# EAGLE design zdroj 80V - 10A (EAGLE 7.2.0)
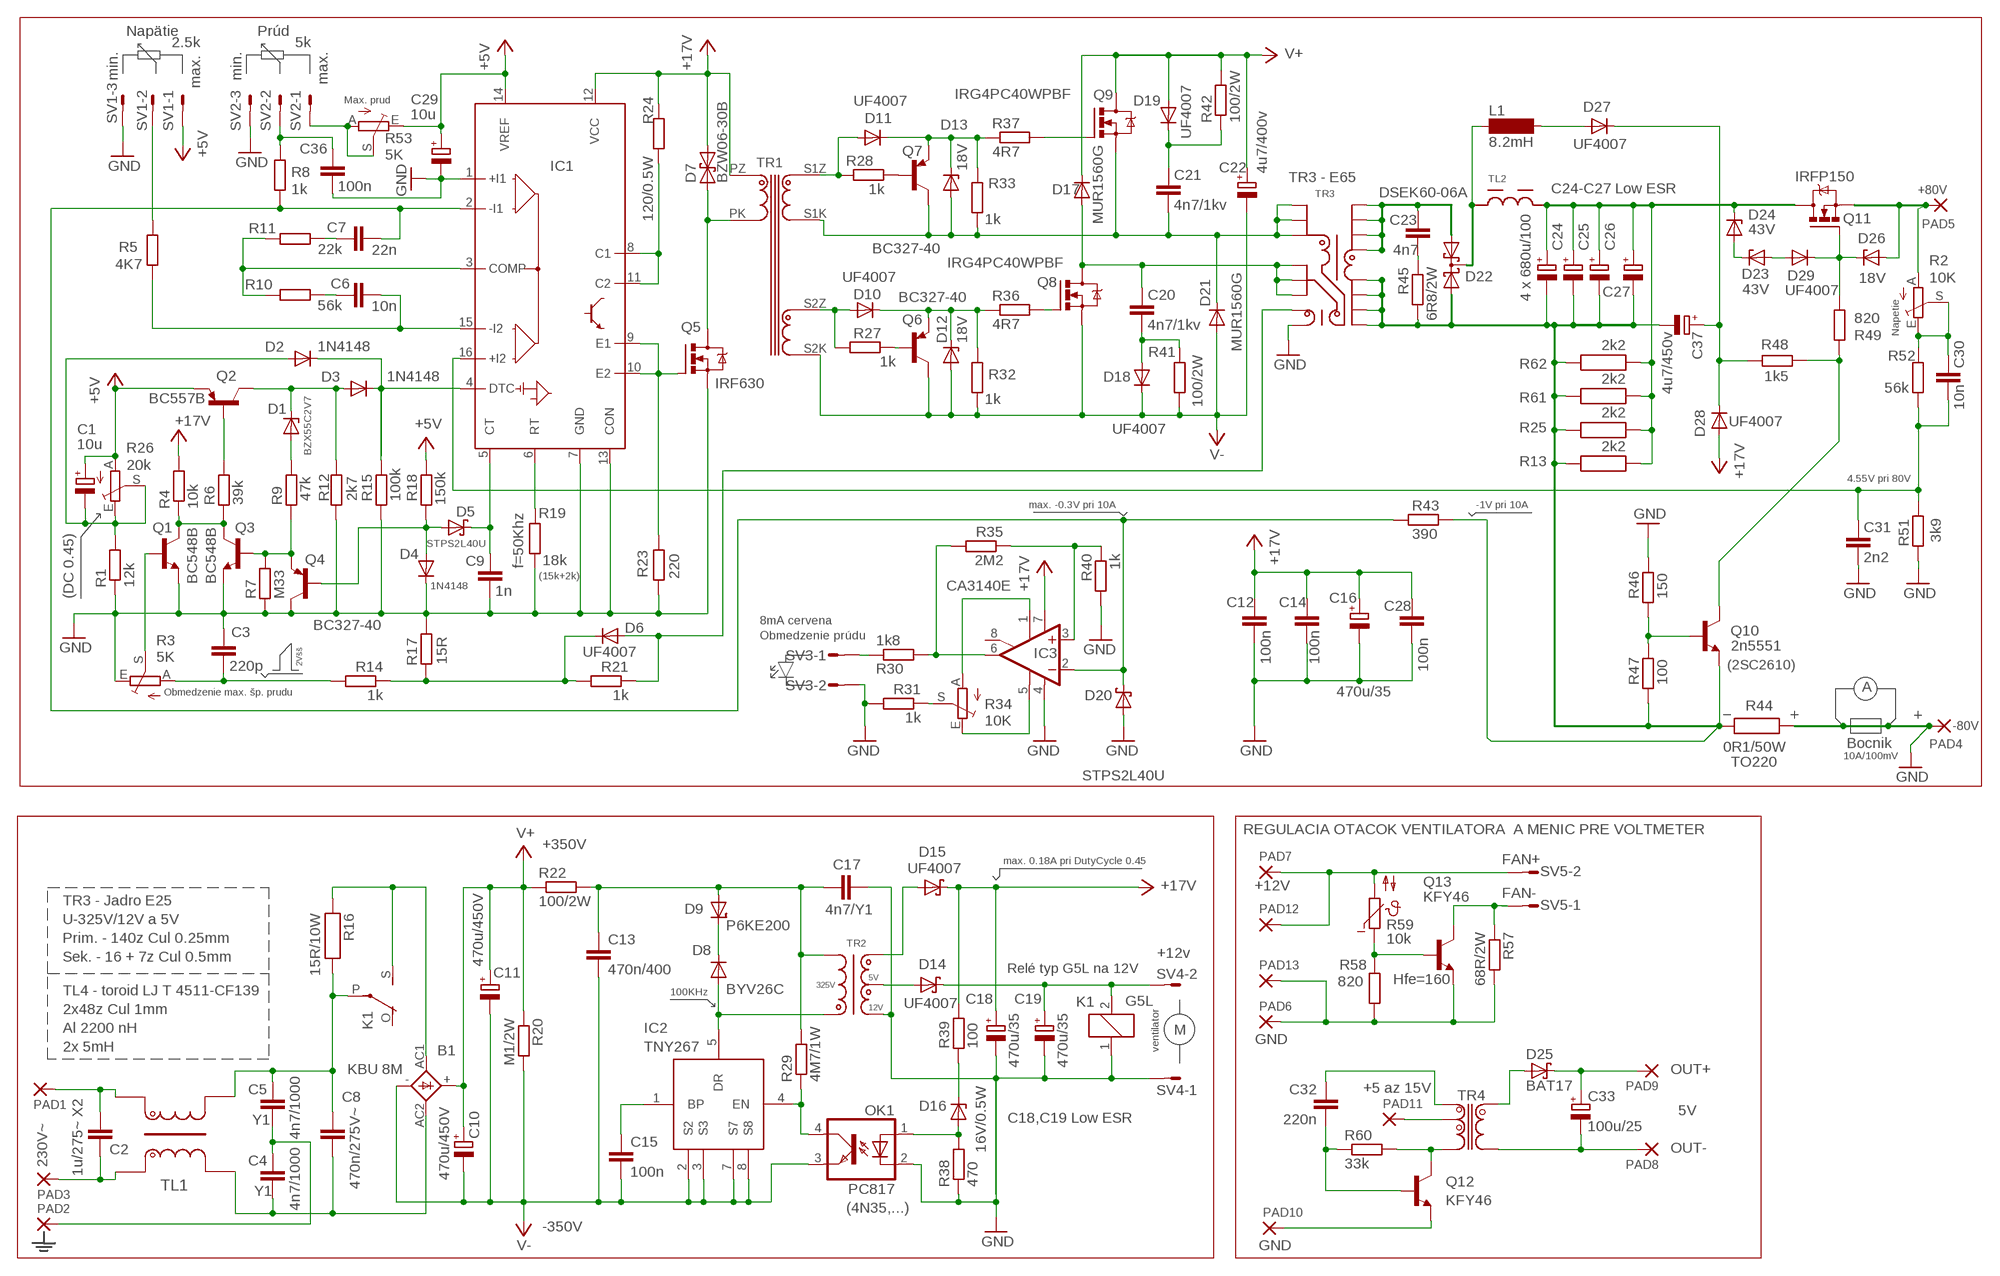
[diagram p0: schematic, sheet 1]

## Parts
B1  KBU 8M  KBU  [KBU]
C1  10u  CPOL-EUE5-4  [E5-4]
C2  1u/275~ X2  C-EU275-134X316  [C275-134X316]
C3  220p  C-EU050-024X044  [C050-024X044]
C4  4n7/1000  C-EU075-032X103  [C075-032X103]
C5  4n7/1000  C-EU075-032X103  [C075-032X103]
C6  10n  C-EU075-032X103  [C075-032X103]
C7  22n  C-EU050-024X044  [C050-024X044]
C8  470n/275V~  FOLIOVYRM22,5/10-26,5  [FOLIOVY_RM22,5/10-26,5]
C9  1n  C-EU050-024X044  [C050-024X044]
C10  470u/450V  CPOL-EUE10-30  [EB30D]
C11  470u/450V  CPOL-EUE10-30  [EB30D]
C12  100n  C-EU050-024X044  [C050-024X044]
C13  470n/400  C-EU225-087X268  [C225-087X268]
C14  100n  C-EU050-024X044  [C050-024X044]
C15  100n  C-EU050-024X044  [C050-024X044]
C16  470u/35  CPOL-EUE5-10.5  [E5-10,5]
C17  4n7/Y1  C-EU075-032X103  [C075-032X103]
C18  470u/35  CPOL-EUE5-10.5  [E5-10,5]
C19  470u/35  CPOL-EUE5-10.5  [E5-10,5]
C20  4n7/1kv  C-EU050-024X044  [C050-024X044]
C21  4n7/1kv  C-EU050-024X044  [C050-024X044]
C22  4u7/400v  CPOL-EUE5-10.5  [E5-10,5]
C23  4n7  C-EU050-024X044  [C050-024X044]
C24  CPOL-EUE7.5-18  [E7,5-18]
C25  CPOL-EUE7.5-18  [E7,5-18]
C26  CPOL-EUE7.5-18  [E7,5-18]
C27  4 x 680u/100  CPOL-EUE7.5-18  [E7,5-18]
C28  100n  C-EU050-024X044  [C050-024X044]
C29  10u  CPOL-EUE2.5-5  [E2,5-5]
C30  10n  C-EU075-032X103  [C075-032X103]
C31  2n2  C-EU050-024X044  [C050-024X044]
C32  220n  C-EU050-024X044  [C050-024X044]
C33  100u/25  CPOL-EUE2.5-6  [E2,5-6]
C36  100n  C-EU050-024X044  [C050-024X044]
C37  4u7/450v  CPOL-EUE5-10.5  [E5-10,5]
D1  BZX55C2V7  ZENER-DIODEDO34-7  [DO34Z7]
D2  1N4148  1N4148DO35-7  [DO35-7]
D3  1N4148  1N4148DO35-7  [DO35-7]
D4  1N4148  1N4148DO35-10  [DO35-10]
D5  STPS2L40U  BAT19  [DO35-10]
D6  UF4007  1N4004  [DO41-10]
D7  BZW06-30B  ZZ22  [P2-15]
D8  BYV26C  DIODE-D-7.5  [D-7.5]
D9  P6KE200  DIODE-DO204-10  [DO204-10]
D10  UF4007  1N4148DO35-7  [DO35-7]
D11  UF4007  1N4148-12  [DO35-12]
D12  18V  BZX90  [DO34Z7]
D13  18V  BZX90  [DO34Z7]
D14  UF4007  BAT49  [DO41-10]
D15  UF4007  BAT49  [DO41-10]
D16  16V/0.5W  BZX90  [DO34Z7]
D17  MUR1560G  BYW29  [DO220S]
D18  UF4007  1N4004  [DO41-10]
D19  UF4007  1N4007-12  [DO41-12]
D20  STPS2L40U  BAT19  [DO35-10]
D21  MUR1560G  BYW29  [DO220S]
D22  DSEK60-06A  DIODE_2SCHOTTKY-SOT93V  [SOT93S]
D23  43V  BZX90  [DO34Z7]
D24  43V  BZX90  [DO34Z7]
D25  BAT17  BAT19  [DO35-10]
D26  18V  BZX85  [DO41Z10]
D27  UF4007  DIODE-DO34-7  [DO34-7]
D28  UF4007  DIODE-DO34-7  [DO34-7]
D29  UF4007  DIODE-DO34-7  [DO34-7]
IC1  TL494  [DIL16]
IC2  TNY267  [DIL7]
IC3  CA3140E  OP07N  [DIL08]
K1  G5L  [G5LE]
L1  8.2mH  SD12K100  [SD12K100]
OK1  PC817  [DIL04]
PAD1  2,54/1,0  [2,54/1,0]
PAD2  2,54/1,0  [2,54/1,0]
PAD3  2,54/1,0  [2,54/1,0]
PAD4  -80V  3,81/1,4  [3,81/1,4]
PAD5  +80V  3,81/1,4  [3,81/1,4]
PAD6  2,54/0,8  [2,54/0,8]
PAD7  2,54/0,8  [2,54/0,8]
PAD8  2,54/0,8  [2,54/0,8]
PAD9  2,54/0,8  [2,54/0,8]
PAD10  2,54/0,8  [2,54/0,8]
PAD11  2,54/0,8  [2,54/0,8]
PAD12  2,54/0,8  [2,54/0,8]
PAD13  2,54/0,8  [2,54/0,8]
Q1  BC548B  BC338  [TO92-EBC]
Q2  BC557B  [TO92-EBC]
Q3  BC548B  BC338  [TO92-EBC]
Q4  BC327-40  [TO92-EBC]
Q5  IRF630  IRF540  [TO220BV]
Q6  BC327-40  BC327  [TO92-EBC]
Q7  BC327-40  BC327  [TO92-EBC]
Q8  IRG4PC40WPBF  IRFPC40  [TO247BV]
Q9  IRG4PC40WPBF  IRFPC40  [TO247BV]
Q10  2n5551  29-NPN-TO92-EBC  [TO92-EBC]
Q11  IRFP150  IRFPC40  [TO247BV]
Q12  KFY46  2N1711  [TO39]
Q13  KFY46  2N1711  [TO39]
R1  12k  R-EU_0207/7  [0207/7]
R2  10K  B64YW  [B64YW]
R3  5K  B64YW  [B64YW]
R4  10k  R-EU_0207/10  [0207/10]
R5  4K7  R-EU_0207/7  [0207/7]
R6  39k  R-EU_0207/7  [0207/7]
R7  M33  R-EU_0207/7  [0207/7]
R8  1k  R-EU_0207/7  [0207/7]
R9  47k  R-EU_0207/7  [0207/7]
R10  56k  R-EU_0207/10  [0207/10]
R11  22k  R-EU_0207/7  [0207/7]
R12  2k7  R-EU_0207/10  [0207/10]
R13  2k2  R5W  [R5W]
R14  1k  R-EU_0207/10  [0207/10]
R15  100k  R-EU_0207/10  [0207/10]
R16  15R/10W  RMNS-10  [RMNS-10]
R17  15R  R-EU_0207/10  [0207/10]
R18  150k  R-EU_0207/7  [0207/7]
R19  18k  R-EU_0207/7  [0207/7]
R20  M1/2W  R-EU_0817/7V  [P0817V]
R21  1k  R-EU_0207/10  [0207/10]
R22  100/2W  R-EU_0411/15  [0411/15]
R23  220  R-EU_0207/10  [0207/10]
R24  120/0.5W  R-EU_0207/7  [0207/7]
R25  2k2  R5W  [R5W]
R26  20k  B64YW  [B64YW]
R27  1k  R-EU_0207/7  [0207/7]
R28  1k  R-EU_0207/12  [0207/12]
R29  4M7/1W  R-EU_0207/10  [0207/10]
R30  1k8  R-EU_0207/7  [0207/7]
R31  1k  R-EU_0207/7  [0207/7]
R32  1k  R-EU_0207/7  [0207/7]
R33  1k  R-EU_0207/7  [0207/7]
R34  10K  B64YW  [B64YW]
R35  2M2  R-EU_0207/7  [0207/7]
R36  4R7  R-EU_0207/7  [0207/7]
R37  4R7  R-EU_0207/7  [0207/7]
R38  470  R-EU_0207/10  [0207/10]
R39  100  R-EU_0207/7  [0207/7]
R40  1k  R-EU_0207/7  [0207/7]
R41  100/2W  R-EU_0411/12  [0411/12]
R42  100/2W  R-EU_0411/12  [0411/12]
R43  390  R-EU_0207/12  [0207/12]
R44  0R1/50W  RMNS-10  [RMNS-10]
R45  6R8/2W  R-EU_0309/12  [0309/12]
R46  150  R-EU_0207/10  [0207/10]
R47  100  R-EU_0207/10  [0207/10]
R48  1k5  R-EU_0207/10  [0207/10]
R49  820  R-EU_0207/10  [0207/10]
R51  3k9  R-EU_0207/7  [0207/7]
R52  56k  R-EU_0207/10  [0207/10]
R53  5K  B64YW  [B64YW]
R57  68R/2W  R-EU_0309/10  [0309/10]
R58  820  R-EU_0207/10  [0207/10]
R59  10k  NTC640  [P640]
R60  33k  R-EU_0207/7  [0207/7]
R61  2k2  R5W  [R5W]
R62  2k2  R5W  [R5W]
SV1  S03P  [S03P]
SV2  S03P  [S03P]
SV3  S02P  [S02P]
SV4  S02P  [S02P]
SV5  S02P  [S02P]
TL1  TR-F  [TR-F]
TL2  TL-TOR20/45  [TL-TOR-40/48]
TR1  TR2  [TR2]
TR2  TR4  [TR4]
TR3  TR1-E65-2  [TR1-E65-2]
TR4  TR-X1  [TR-X1]

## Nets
+5V: C1.+ C29.+ IC1.14(VREF) Q2.E R18.1 R26.A R53.E SV1.1
+17V: C12.1 C14.1 C16.+ C18.+ C28.1 D7.C D15.C D28.A IC1.12(VCC) IC3.7(V+) R4.2 R24.1 R39.2 TR1.PZ
GND: C3.2 C9.1 C12.2 C14.2 C16.- C17.2 C18.- C19.- C28.2 C29.- C31.2 C36.2 D4.C D20.A IC1.1(+I1) IC1.7(GND) IC1.13(CON) IC3.4(V-) K1.1 OK1.2(C) PAD4.1(P) Q1.E Q3.E Q4.C Q5.S R1.1 R3.E R7.2 R12.1 R15.1 R17.1 R19.1 R23.2 R31.2 R38.1 R40.2 R44.2 R46.2 R51.1 SV1.3 SV2.3 SV3.2 SV4.1 TR2.P3 TR3.1
N$1: C2.1 PAD3.1(P) TL1.A1
N$2: C2.2 PAD1.1(P) TL1.B1
N$3: C5.1 C8.P$1 K1.P(2:P) R16.2 TL1.B2
N$4: C13.1 C17.1 D9.A R22.2 R29.2 TR2.P1
N$5: C19.+ D14.C K1.2 SV4.2
N$6: B1.AC1 K1.S(2:S) R16.1
N$7: D2.C D3.C IC1.4(DTC) R15.2
N$8: D14.A TR2.P4
N$9: D27.A L1.2
N$10: IC1.9(E1) IC1.10(E2) Q5.G R23.1
N$11: D26.C D29.C Q11.G R49.2
N$13: IC3.3(+IN) R35.1 R40.1
N$14: D26.A PAD5.1(P) Q11.S R2.A
N$15: D8.C D9.C
N$16: C30.1 R2.E R2.S R52.1
N$17: C30.2 C31.1 IC1.16(+I2) R51.2 R52.2
N$18: C9.2 D5.C IC1.5(CT)
N$19: IC1.6(RT) R19.2
N$20: D6.C R14.1 R17.2 R21.2
N$21: D6.A R21.1 TR3.2
N$22: IC1.8(C1) IC1.11(C2) R24.2
N$23: D7.A Q5.D TR1.PK
N$24: Q7.B R28.2
N$25: D23.C D24.A
N$26: D11.A R28.1 TR1.S1Z
N$27: D11.C D13.C Q7.E R33.1 R37.1
N$28: Q6.B R27.2
N$29: D10.A R27.1 TR1.S2Z
N$30: C21.2 D13.A D21.C Q7.C Q9.S R33.2 TR1.S1K TR3.6 TR3.7 TR3.8
N$31: D10.C D12.C Q6.E R32.1 R36.1
N$32: B1.AC2 C4.2 C8.P$2 TL1.A2
N$33: D8.A IC2.5(DR) TR2.P2
N$34: C15.1 IC2.1(BP)
N$35: IC2.4(EN) OK1.4(COL) R29.1
N$36: D22.C L1.1 TL2.2
N$37: D15.A TR2.P5
N$38: Q8.G R36.2
N$39: C20.2 D17.A Q8.D TR3.3 TR3.4 TR3.5
N$40: D16.A OK1.1(A) R38.2
N$41: D16.C R39.1
N$42: Q9.G R37.2
N$43: C1.- D2.A R1.2 R26.E R26.S
N$44: C20.1 D18.A R41.1
N$45: C21.1 D19.C R42.1
N$46: IC3.6(OUT) R30.2 R35.2
N$47: C23.2 D22.A2 TR3.9 TR3.10 TR3.11 TR3.12
N$48: C24.+ C25.+ C26.+ C27.+ D24.C Q11.D R13.1 R25.1 R61.1 R62.1 TL2.1
N$49: C7.2 D20.C IC1.2(-I1) IC3.2(-IN) R8.2 R43.1
N$50: D1.C D3.A Q2.C R12.2
N$51: C24.- C25.- C26.- C27.- C37.- D22.A1 Q10.E R13.2 R25.2 R43.2 R44.1 R45.2 R47.1 R61.2 R62.2 TR3.13 TR3.14 TR3.15 TR3.16
N$52: R53.A R53.S SV2.1
N$53: C36.1 R8.1 SV2.2
N$54: C6.2 IC1.15(-I2) R5.1
N$55: R5.2 SV1.2
N$56: Q10.B R46.1 R47.2
N$57: PAD7.1(P) PAD12.1(P) R59.2 SV5.2
N$58: C6.1 R10.2
N$59: Q2.B R6.1
N$60: PAD6.1(P) PAD13.1(P) Q13.1(E) R57.2 R58.1
N$61: Q1.C Q3.C R4.1 R6.2
N$62: Q13.3(C) R57.1 SV5.1
N$63: Q3.B Q4.E R7.1 R9.2
N$64: IC3.5(OPT) R34.E
N$65: IC3.1(ON1) R34.A
N$66: IC1.3(COMP) R10.1 R11.1
N$67: Q10.C R48.2 R49.1
N$68: R31.1 R34.S
N$69: C7.1 R11.2
N$70: C37.+ D27.C D28.C R48.1
N$71: C3.1 R3.A R14.2
N$72: C4.1 C5.2 PAD2.1(P)
N$73: Q1.B R3.S
N$74: R30.1 SV3.1
N$75: Q13.2(B) R58.2 R59.1
N$76: C32.2 Q12.2(B) R60.1
N$77: Q12.3(C) R60.2 TR4.P
N$78: C33.+ D25.C PAD9.1(P)
N$79: D1.A R9.1
N$80: D4.A D5.A Q4.B R18.2
N$81: C23.1 R45.1
N$82: C33.- PAD8.1(P) TR4.S2
N$83: C32.1 TR4.I(B)
N$84: PAD11.1(P) TR4.SP
N$85: PAD10.1(P) Q12.1(E)
N$86: D25.A TR4.S1
N$93: D23.A D29.A
V+: B1.+ C10.+ C11.+ C22.+ D17.C D19.A Q9.D R20.1 R22.1 R42.2
V-: B1.- C10.- C11.- C13.2 C15.2 C22.- D12.A D18.C D21.A IC2.2(S2) IC2.3(S3) IC2.7(S7) IC2.8(S8) OK1.3(EMIT) Q6.C Q8.S R20.2 R32.2 R41.2 TR1.S2K
Unconnected: IC3.8(ON2) K1.O(2:O)

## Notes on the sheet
- Napätie | Prúd
- min. | 2.5k | min. | 5k | max.
- max.
- Max. prud
- TR3 - E65
- C24-C27 Low ESR
- Napetie
- 4.55V pri 80V
- max. -0.3V pri 10A | -1V pri 10A
- f=50Khz
- (15k+2k)
- (DC 0.45)
- 8mA cervena
- Obmedzenie prúdu
- 2Všš
- (2SC2610)
- A
- Obmedzenie max. šp. prudu
- Bocnik
- 10A/100mV
- TO220
- REGULACIA OTACOK VENTILATORA  A MENIC PRE VOLTMETER
- +350V
- max. 0.18A pri DutyCycle 0.45 | FAN+
- +12V
- FAN-
- TR3 - Jadro E25
- U-325V/12V a 5V
- Prim. - 140z Cul 0.25mm
- Sek. - 16 + 7z Cul 0.5mm | +12v
- Relé typ G5L na 12V
- 5V
- Hfe=160
- 325V
- TL4 - toroid LJ T 4511-CF139 | 100KHz
- 12V
- 2x48z Cul 1mm
- Al 2200 nH | M
- GND
- 2x 5mH | ventilator
- OUT+
- +5 az 15V
- 5V
- 230V~ | Y1 | C18,C19 Low ESR
- OUT-
- Y1
- (4N35,...)
- -350V
- GND

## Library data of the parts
B1 = rectifier:KBU: DIOTEC RECTIFIER
C1 C10 C11 C16 C18 C19 C22 C24-C27 C29 C33 C37 = rcl:CPOL-EU: POLARIZED CAPACITOR, European symbol
C2-C7 C9 C12-C15 C17 C20 C21 C23 C28 C30-C32 C36 = rcl:C-EU: CAPACITOR, European symbol
C8 = #Kondenzatory:FOLIOVY
D1 = diode:ZENER-DIODE: Z-Diode
D2-D4 D10 = diode:1N4148: DIODE
D5 D20 D25 = diode:BAT19: DIODE
D6 D18 = diode:1N4004: DIODE
D7 = diode:ZZ22: DIODE
D8 D9 D27-D29 = diode:DIODE-: DIODE
D11 = diode-1:1N4148-12
D12 D13 D16 D23 D24 = diode:BZX90: Z DIODE
D14 D15 = diode:BAT49: DIODE
D17 D21 = diode:BYW29: DIODE
D19 = UNIVERSAL:1N4007-12
D22 = diode-1:DIODE_2SCHOTTKY-: Dual SCHOTTKY DIODE common cathode
D26 = diode:BZX85: Z DIODE
IC1 = UNIVERSAL:TL494: TL494N upraveny pre priepustny menic. DIL16
IC2 = UNIVERSAL:TNY267; IC: TNY267
IC3 = linear:OP07*: OP AMP
K1 = relay:G5L: RELAY 1 x switch, 10 A/120 V AC, 8 A/30 V ADC, Omron
L1 = inductor-neosid:SD12: INDUCTOR; OC_FARNELL: unknown; OC_NEWARK: unknown
OK1 = optocoupler:PC817: SHARP OPTO COUPLER; MPN: PC817X4J000F; OC_FARNELL: 9707727; OC_NEWARK: 97K7059
PAD1-PAD3 = PLOSNE BODY:2,54/1,0
PAD4 PAD5 = PLOSNE BODY:3,81/1,4
PAD6-PAD13 = PLOSNE BODY:2,54/0,8
Q1 Q3 = transistor-npn:BC338*: NPN Transistor
Q2 = transistor-pnp:BC557*: PNP Transistror
Q4 Q6 Q7 = transistor-pnp:BC327*: PNP Transistror
Q5 = transistor-power:IRF540: HEXFET Power MOSFET
Q8 Q9 Q11 = transistor-power:IRFPC40: N-CHANNEL MOS FET
Q10 = transistor:*-NPN-: NPN Transistror BF959 corrected 2008.03.06
Q12 Q13 = transistor-npn:2N1711: NPN Transistor
R1 R4-R12 R14 R15 R17-R24 R27-R33 R35-R43 R45-R49 R51 R52 R57 R58 R60 = rcl:R-EU_: RESISTOR, European symbol
R2 R3 R26 R34 R53 = pot:B64YW
R13 R25 R61 R62 = UNIVERSAL:R5W
R16 R44 = UNIVERSAL:RMNS-10
R59 = ptc-ntc:NTC640: PHILIPS NTC; OC_FARNELL: unknown; OC_NEWARK: unknown
SV1 SV2 = con-amp-mt:S03P: AMP MT CONNECTOR; OC_FARNELL: unknown; OC_NEWARK: unknown
SV3-SV5 = con-amp-mt:S02P: AMP MT CONNECTOR; OC_FARNELL: unknown; OC_NEWARK: unknown
TL1 = UNIVERSAL:TR-F
TL2 = UNIVERSAL:TL-TOR20/45
TR1 = UNIVERSAL:TR2
TR2 = UNIVERSAL:TR4
TR3 = UNIVERSAL:TR1-E65-2: Trafo E65 s prehodenymi vyvodami.
TR4 = UNIVERSAL:TR-X1

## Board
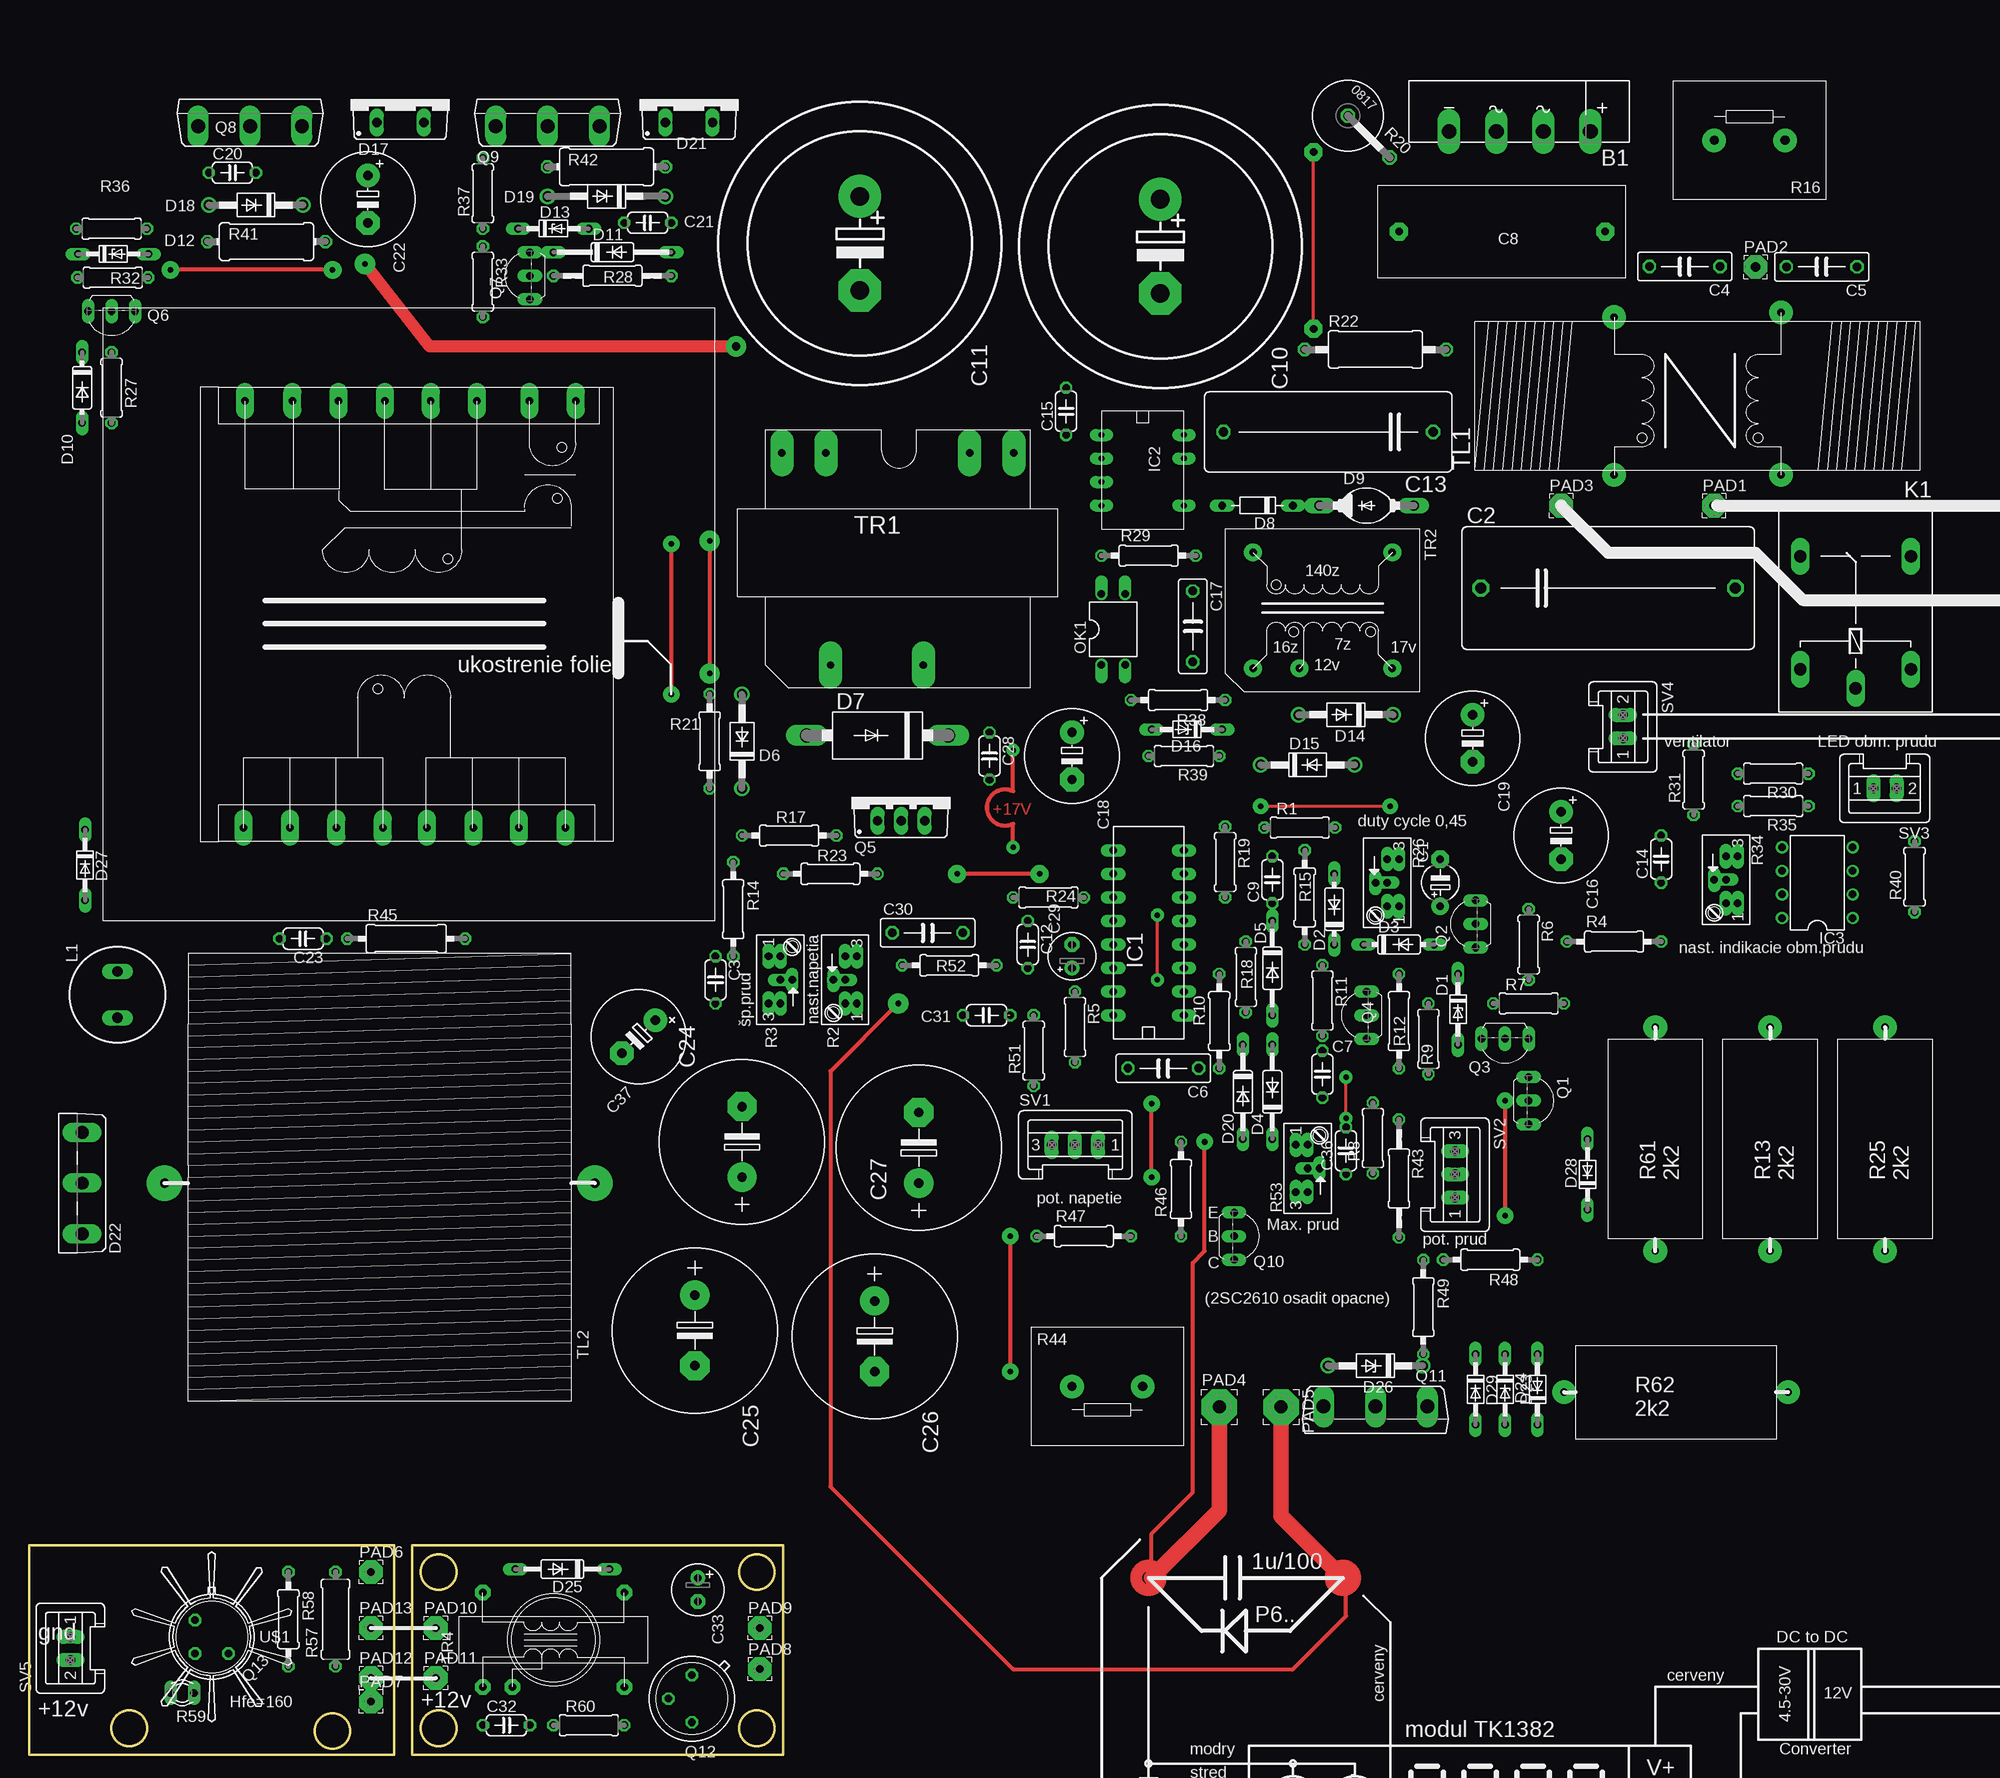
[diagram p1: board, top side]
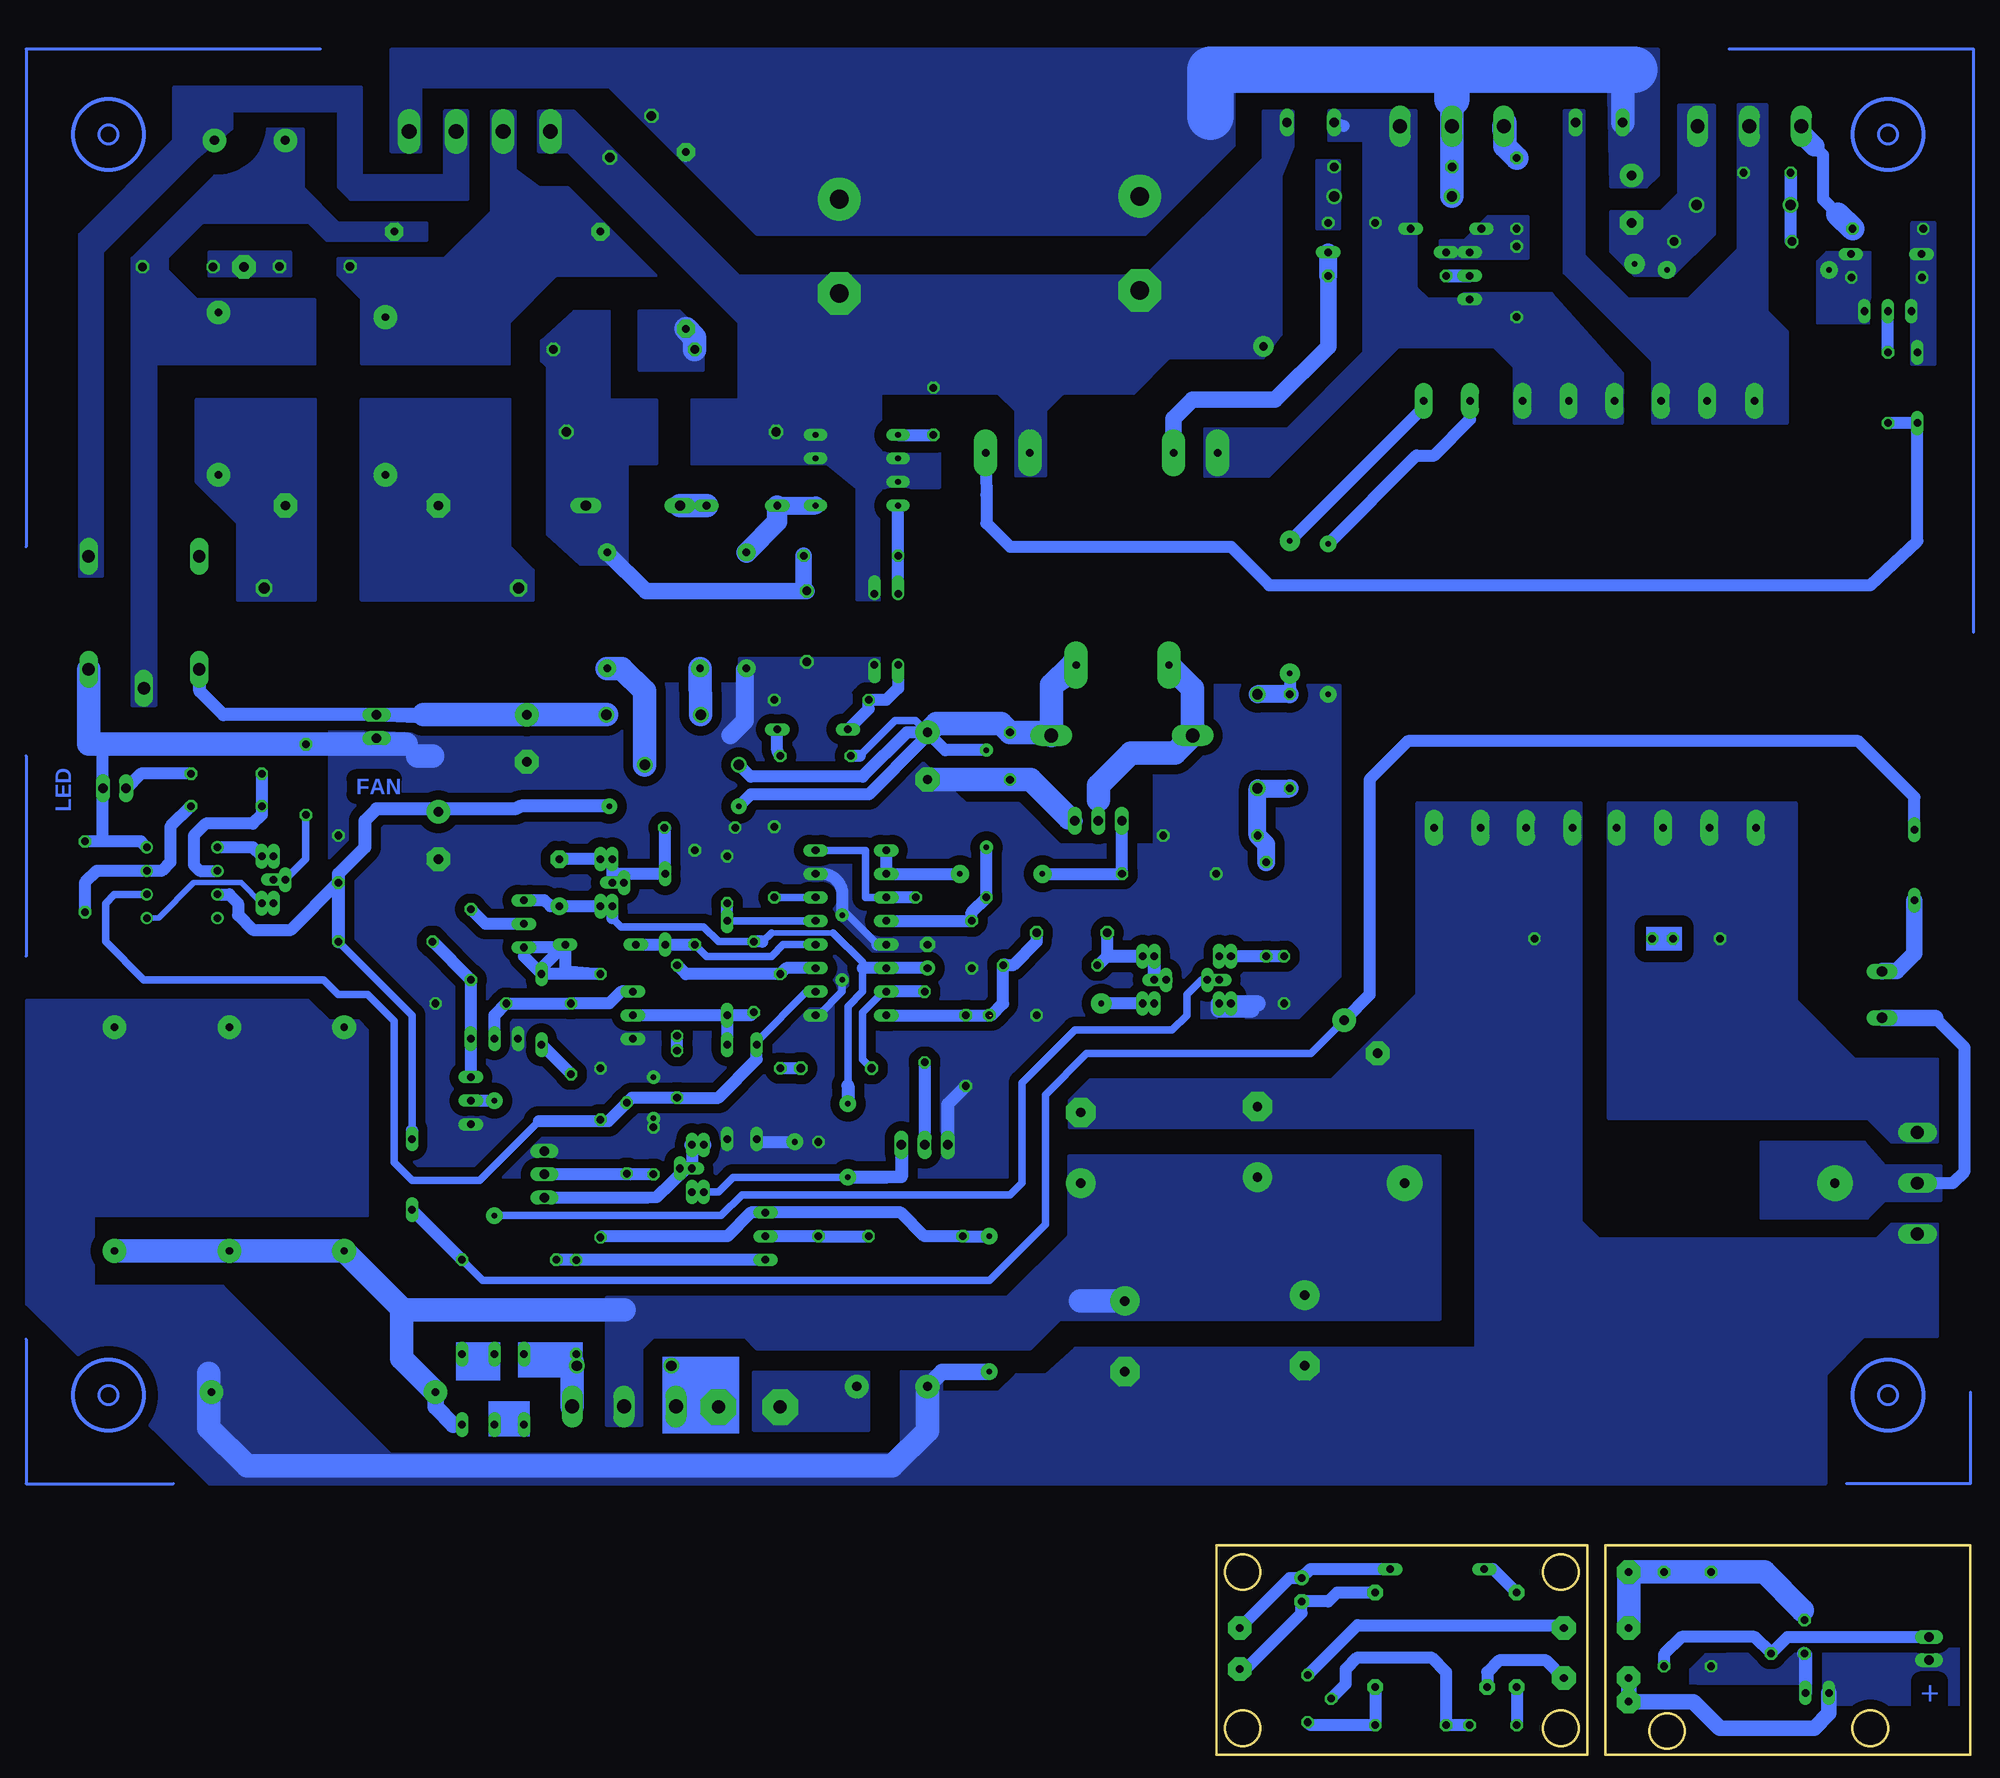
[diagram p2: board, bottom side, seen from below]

Size 81.28 x 22.54 mm. Coordinates in mm from the lower left corner, seen from the top.
Outline: 0,0 39.37,0 39.37,22.54 0,22.54 0,0
Outline: 41.27,0 41.27,22.54 81.28,22.54 81.28,0 41.27,0
Outline: circle at 10.79,2.86 radius 1.91
Outline: circle at 32.7,2.54 radius 1.91
Outline: circle at 44.13,2.86 radius 1.91
Outline: circle at 44.13,19.69 radius 1.91
Outline: circle at 78.42,19.69 radius 1.91
Outline: circle at 78.42,2.86 radius 1.91
Copper layers (1*16): Top 0.035mm / dielectric 1.5mm / Bottom 0.035mm
Design rules "default": minimum track width 10mil, minimum drill 24mil, track to track 8mil, track to pad 8mil, pad to pad 8mil, via to via 8mil, smd to smd 8mil, copper to edge 40mil, drill to drill 8mil, minimum pad ring 10mil, minimum via ring 8mil, stop-mask expansion 4mil, vias tented up to drill 0mil, thermal gap 10mil

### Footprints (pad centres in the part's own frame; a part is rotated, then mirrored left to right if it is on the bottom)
KBU = drill 1.6 long: + -7.62,2.54; - 7.62,2.54; AC1 -2.54,2.54; AC2 2.54,2.54
E5-4 = drill 0.813 pad 1.905: + -2.54,0 | drill 0.813 pad 1.905 octagon: - 2.54,0
C275-134X316 = drill 1.194 octagon: 1 -13.716,0; 2 13.716,0
C050-024X044 = drill 0.813 octagon: 1 -2.54,0; 2 2.54,0
C075-032X103 = drill 0.914 octagon: 1 -3.81,0; 2 3.81,0
FOLIOVY_RM22,5/10-26,5 = drill 0.8 pad 1.93 octagon: P$1 -11.113,0; P$2 11.113,0
EB30D = drill 2.007 pad 4.597: + -5.08,0 | drill 2.007 pad 4.597 octagon: - 5.08,0
C225-087X268 = drill 1.016 octagon: 1 -11.303,0; 2 11.303,0
E5-10,5 = drill 1.016 pad 2.54: + -2.54,0 | drill 1.016 pad 2.54 octagon: - 2.54,0
E7,5-18 = drill 1.016 pad 3.15: + -3.81,0 | drill 1.016 pad 3.15 octagon: - 3.81,0
E2,5-5 = drill 0.813 pad 1.6: + -1.27,0 | drill 0.813 pad 1.6 octagon: - 1.27,0
E2,5-6 = drill 0.813 pad 1.6: + -1.27,0 | drill 0.813 pad 1.6 octagon: - 1.27,0
DO34Z7 = drill 0.813 long: A 3.81,0; C -3.81,0
DO35-7 = drill 0.813 long: A 3.81,0; C -3.81,0
DO35-10 = drill 0.813 long: A 5.08,0; C -5.08,0
DO41-10 = drill 1.118: A 5.08,0; C -5.08,0
P2-15 = drill 1.499 long: A 7.62,0; C -7.62,0
D-7.5 = drill 0.813 long: A 3.81,0; C -3.81,0
DO204-10 = drill 1.118 long: A 5.08,0; C -5.08,0
DO35-12 = drill 0.813 long: A 6.35,0; C -6.35,0
DO220S = drill 1.016 long: A 2.54,-2.54; C -2.54,-2.54
DO41-12 = drill 1.118: A 6.35,0; C -6.35,0
SOT93S = drill 1.397 long: A1 -5.461,-2.54; A2 5.461,-2.54; C 0,-2.54
DO41Z10 = drill 1.118: A 5.08,0; C -5.08,0
DO34-7 = drill 0.813 long: A 3.81,0; C -3.81,0
DIL16 = drill 0.813 pad 1.27 long: 1 0,1.27; 2 2.54,1.27; 3 5.08,1.27; 4 7.62,1.27; 5 10.16,1.27; 6 12.7,1.27; 7 15.24,1.27; 8 17.78,1.27; 9 17.78,8.89; 10 15.24,8.89; 11 12.7,8.89; 12 10.16,8.89; 13 7.62,8.89; 14 5.08,8.89; 15 2.54,8.89; 16 0,8.89
DIL7 = drill 0.61 pad 1.27 long: 1 2.54,0; 2 5.08,0; 3 7.62,0; 4 10.16,0; 5 10.16,8.89; 7 5.08,8.89; 8 2.54,8.89
DIL08 = drill 0.813 pad 1.27: 1 -3.81,-3.81; 2 -1.27,-3.81; 3 1.27,-3.81; 4 3.81,-3.81; 5 3.81,3.81; 6 1.27,3.81; 7 -1.27,3.81; 8 -3.81,3.81
G5LE = drill 1.321 long: 1 -7.493,-5.969; 2 -7.493,5.969; O 4.699,5.969; P -9.525,0; S 4.699,-5.969
SD12K100 = drill 1.1 long: 1 -2.5,0; 2 2.5,0
DIL04 = drill 0.813 offset: 1 -1.27,-3.81; 2 1.27,-3.81; 3 1.27,3.81; 4 -1.27,3.81
2,54/1,0 = drill 1.016 pad 2.54 octagon: 1 0,0
3,81/1,4 = drill 1.397 pad 3.81 octagon: 1 0,0
2,54/0,8 = drill 0.813 pad 2.54 octagon: 1 0,0
TO92-EBC = drill 0.813 long: B 0,-1.27; C -2.54,-1.27; E 2.54,-1.27
TO220BV = drill 1.016 long: D 0,-2.54; G -2.54,-2.54; S 2.54,-2.54
TO247BV = drill 1.499 long: D 0,-2.921; G -5.588,-2.921; S 5.588,-2.921
TO92-EBC' = drill 0.813 long: B 0,-1.27; C 2.54,-1.27; E -2.54,-1.27
TO39 = drill 0.813 octagon: 1 0,-2.54; 2 2.54,0; 3 0,2.54
0207/7 = drill 0.813 octagon: 1 -3.81,0; 2 3.81,0
B64YW = drill 0.813 long: A 2.54,0; A1 2.54,1.27; E -2.54,0; E1 -2.54,1.27; S 0,0; S1 0,-1.27 | drill 0.813 octagon: S2 0,-1.27
0207/10 = drill 0.813 octagon: 1 -5.08,0; 2 5.08,0
R5W = drill 0.8 pad 2.54: 1 1.27,0; 2 25.4,0
RMNS-10 = drill 1 pad 2.54: 1 4.445,6.35; 2 12.065,6.35
P0817V = drill 1.016 octagon: 1 -5.08,0; 2 1.27,0
0411/15 = drill 0.914 octagon: 1 -7.62,0; 2 7.62,0
0207/12 = drill 0.813 octagon: 1 -6.35,0; 2 6.35,0
0411/12 = drill 0.914 octagon: 1 -6.35,0; 2 6.35,0
0309/12 = drill 0.813 octagon: 1 -6.35,0; 2 6.35,0
0309/10 = drill 0.813 octagon: 1 -5.08,0; 2 5.08,0
P640 = drill 0.813 long: 1 -1.27,0; 2 1.27,0
S03P = drill 1.016 long: 1 2.5,0; 2 0,0; 3 -2.5,0
S02P = drill 1.016 long: 1 1.25,0; 2 -1.25,0
TR-F = drill 0.8 pad 2.54: A1 -0.5,33; A2 16.5,33; B1 -0.5,15; B2 17,15
TL-TOR-40/48 = drill 1 pad 3.81: 1 -2.54,24.765; 2 43.815,24.765
TR2 = drill 0.8 pad 2.54 long: PK 7,3.135; PZ 17,3.135; S1K 1.75,26; S1Z 6.5,26; S2K 22,26; S2Z 26.75,26
TR4 = drill 0.8 pad 1.93: P1 2.5,18; P2 2.5,3; P3 15,3; P4 15,8; P5 15,18
TR1-E65-2 = drill 0.8 pad 1.93 long: 1 10,-20.06; 2 10,-15.06; 3 10,-50.7; 4 10,-45.62; 5 10,-40.62; 6 10,-35.62; 7 10,-30.7; 8 10,-25.7; 9 56,-35.86; 10 56,-40.86; 11 56,-45.86; 12 56,-50.86; 13 56,-16.172; 14 56,-21.172; 15 56,-26.093; 16 56,-31.093
TR-X1 = drill 0.8 pad 1.676 octagon: I -2.54,17.78; P -2.54,2.54; S1 7.62,17.78; S2 7.62,2.54; SP -2.54,14.605

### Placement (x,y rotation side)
B1  not placed on the board
C1  152.08,93.98 90 top  (outside the outline)
C2  not placed on the board
C3  73.98,83.5 270 top  (outside the outline)
C4  not placed on the board
C5  not placed on the board
C6  122.24,73.98 180 top  (outside the outline)
C7  139.38,73.34 270 top  (outside the outline)
C8  not placed on the board
C9  133.99,94.3 270 top  (outside the outline)
C10  not placed on the board
C11  not placed on the board
C12  107.63,87.31 270 top  (outside the outline)
C13  not placed on the board
C14  175.9,96.52 90 top  (outside the outline)
C15  111.76,144.78 90 top  (outside the outline)
C16  165.1,99.06 270 top  (outside the outline)
C17  125.41,121.6 270 top  (outside the outline)
C18  112.39,107.63 270 top  (outside the outline)
C19  155.58,109.54 270 top  (outside the outline)
C20  21.91,170.5 0 top  (outside the outline)
C21  not placed on the board
C22  not placed on the board
C23  29.53,87.95 180 top  (outside the outline)
C24  not placed on the board
C25  not placed on the board
C26  91.12,45.09 270 top  (outside the outline)
C27  not placed on the board
C28  103.5,107.63 270 top  (outside the outline)
C29  112.39,86.04 90 top  (outside the outline)
C30  96.84,88.58 0 top  (outside the outline)
C31  not placed on the board
C32  51.44,3.18 0 top
C33  72.07,17.78 270 top
C36  141.92,65.09 90 top  (outside the outline)
C37  65.68,77.38 225 top  (outside the outline)
D1  153.99,80.33 270 top  (outside the outline)
D2  140.65,91.12 90 top  (outside the outline)
D3  147.64,87.31 0 top  (outside the outline)
D4  133.99,71.44 90 top  (outside the outline)
D5  133.99,84.77 270 top  (outside the outline)
D6  76.83,109.22 90 top  (outside the outline)
D7  91.44,109.85 180 top  (outside the outline)
D8  132.4,134.62 180 top  (outside the outline)
D9  144.15,134.62 0 top  (outside the outline)
D10  5.71,147.32 270 top  (outside the outline)
D11  62.87,161.93 0 top  (outside the outline)
D12  not placed on the board
D13  not placed on the board
D14  141.92,112.08 180 top  (outside the outline)
D15  137.8,106.68 0 top  (outside the outline)
D16  124.78,110.49 180 top  (outside the outline)
D17  40.01,178.44 0 top  (outside the outline)
D18  24.45,167 180 top  (outside the outline)
D19  62.23,167.96 180 top  (outside the outline)
D20  130.81,71.44 270 top  (outside the outline)
D21  71.12,178.44 0 top  (outside the outline)
D22  3.17,61.59 90 top  (outside the outline)
D23  159.07,39.37 270 top  (outside the outline)
D24  162.56,39.37 90 top  (outside the outline)
D25  57.47,20 180 top
D26  145.1,41.91 180 top  (outside the outline)
D27  6.03,95.88 270 top  (outside the outline)
D28  167.96,62.55 90 top  (outside the outline)
D29  155.89,39.37 270 top  (outside the outline)
IC1  125.73,79.69 90 top  (outside the outline)
IC2  115.57,144.78 270 top  (outside the outline)
IC3  192.72,93.98 90 top  (outside the outline)
K1  196.85,124.46 90 top  (outside the outline)
L1  9.53,81.91 90 top  (outside the outline)
OK1  116.84,121.28 0 top  (outside the outline)
PAD1  not placed on the board
PAD2  not placed on the board
PAD3  not placed on the board
PAD4  128.27,37.47 0 top  (outside the outline)
PAD5  134.94,37.47 270 top  (outside the outline)
PAD6  36.83,19.69 0 top
PAD7  36.83,5.71 0 top
PAD8  78.74,9.21 0 top
PAD9  78.74,13.65 0 top
PAD10  43.82,13.65 0 top
PAD11  43.82,8.26 0 top
PAD12  36.83,8.26 0 top
PAD13  36.83,13.65 0 top
Q1  162.88,70.48 270 top  (outside the outline)
Q2  154.62,89.53 90 top  (outside the outline)
Q3  159.07,75.88 180 top  (outside the outline)
Q4  142.88,79.69 90 top  (outside the outline)
Q5  93.98,103.19 0 top  (outside the outline)
Q6  8.89,154.31 180 top  (outside the outline)
Q7  52.71,159.39 90 top  (outside the outline)
Q8  23.81,178.44 0 top  (outside the outline)
Q9  55.88,178.44 0 top  (outside the outline)
Q10  2n5551  [TO92-EBC']  131.13,55.88 270 top  (outside the outline)
Q11  145.1,34.61 180 top  (outside the outline)
Q12  71.44,6.03 180 top
Q13  19.68,12.7 225 top
R1  136.94,99.92 0 top  (outside the outline)
R2  87.95,83.5 270 top  (outside the outline)
R3  80.96,83.5 90 top  (outside the outline)
R4  170.81,87.63 0 top  (outside the outline)
R5  112.71,78.42 270 top  (outside the outline)
R6  161.61,87.31 270 top  (outside the outline)
R7  161.61,80.96 0 top  (outside the outline)
R8  144.82,66.45 90 top  (outside the outline)
R9  150.81,77.15 90 top  (outside the outline)
R10  128.27,79.06 270 top  (outside the outline)
R11  139.38,81.28 270 top  (outside the outline)
R12  147.64,79.06 90 top  (outside the outline)
R13  187.64,53.02 90 top  (outside the outline)
R14  75.88,91.12 270 top  (outside the outline)
R15  137.48,92.39 270 top  (outside the outline)
R16  not placed on the board
R17  81.91,99.06 180 top  (outside the outline)
R18  131.13,83.82 270 top  (outside the outline)
R19  128.91,96.2 270 top  (outside the outline)
R20  not placed on the board
R21  73.34,109.22 270 top  (outside the outline)
R22  145.1,151.45 0 top  (outside the outline)
R23  86.36,94.93 180 top  (outside the outline)
R24  109.85,92.39 0 top  (outside the outline)
R25  200.03,53.02 90 top  (outside the outline)
R26  146.37,93.98 270 top  (outside the outline)
R27  8.89,147.32 90 top  (outside the outline)
R28  62.87,159.39 180 top  (outside the outline)
R29  120.65,129.22 0 top  (outside the outline)
R30  187.96,105.73 180 top  (outside the outline)
R31  179.39,105.09 90 top  (outside the outline)
R32  not placed on the board
R33  not placed on the board
R34  182.88,94.3 270 top  (outside the outline)
R35  187.96,102.24 180 top  (outside the outline)
R36  8.89,164.47 0 top  (outside the outline)
R37  48.9,168.28 90 top  (outside the outline)
R38  123.82,113.66 180 top  (outside the outline)
R39  124.46,107.63 180 top  (outside the outline)
R40  203.2,94.62 90 top  (outside the outline)
R41  25.59,163.06 0 top  (outside the outline)
R42  62.23,171.13 180 top  (outside the outline)
R43  147.64,62.1 270 top  (outside the outline)
R44  107.95,33.34 0 top  (outside the outline)
R45  40.64,87.95 0 top  (outside the outline)
R46  124.14,60.96 90 top  (outside the outline)
R47  113.66,55.88 0 top  (outside the outline)
R48  157.48,53.34 180 top  (outside the outline)
R49  150.26,48.24 270 top  (outside the outline)
R51  108.27,75.88 90 top  (outside the outline)
R52  99.17,85.07 0 top  (outside the outline)
R53  137.8,63.18 90 top  (outside the outline)
R57  33.02,14.61 90 top
R58  27.94,14.61 270 top
R59  16.51,6.67 180 top
R60  60.33,3.18 0 top
R61  175.26,53.02 90 top  (outside the outline)
R62  164.15,39.05 0 top  (outside the outline)
SV1  112.71,65.72 0 top  (outside the outline)
SV2  153.67,62.55 270 top  (outside the outline)
SV3  200.03,104.14 180 top  (outside the outline)
SV4  171.77,110.81 270 top  (outside the outline)
SV5  4.45,11.43 90 top
TL1  not placed on the board
TL2  not placed on the board
TR1  79.38,114.3 0 top  (outside the outline)
TR2  128.91,132.08 270 top  (outside the outline)
TR3  73.98,155.89 270 top  (outside the outline)
TR4  66.67,9.84 90 top
U$1  [KK505]  19.68,12.7 0 top

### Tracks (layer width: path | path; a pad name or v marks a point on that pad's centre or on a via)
+5V  (via drill 0.6 pad 1.78)
  Top 0.406: v120.97,62.23 v120.97,70.17
  Bottom 0.61: 122.55,88.58 129.22,88.58
  Bottom 0.813: 122.55,88.58 119.38,85.41 119.38,84.77 119.38,82.23 120.97,80.65 120.97,72.07 | 129.22,88.58 130.18,87.63 | R18.1 134.94,87.63 136.53,89.22 145.42,89.22 146.37,90.17 | R53.E 134.94,60.64 133.35,62.23 v120.97,62.23
  Bottom 1.27: 119.38,84.77 IC1.14 C29.+ | Q2.E 153.67,92.08 153.03,91.44 C1.+ R26.A 146.37,90.17 | 130.18,87.63 R18.1
  Bottom 1.422: 120.97,72.07 v120.97,70.17 | SV1.1 115.21,62.27 116.84,62.23 v120.97,62.23
+17V  (via drill 0.6 pad 1.42, 0.6 pad 1.68)
  Top 0.305: v132.72,102.24 v146.69,102.24
  Top 0.406: v106.05,97.79 106.05,100.33 arc-233 106.05,103.82 v106.05,108.27
  Bottom 0.61: C16.+ 167.32,101.92
  Bottom 0.813: 167.96,67.31 167.96,79.69 R4.2 | 119.7,107.63 115.89,111.44 113.66,111.44 C18.+
  Bottom 1.27: C18.+ 114.62,110.17 119.38,105.41 131.45,105.41 D15.C | v132.72,102.24 131.45,103.5 118.74,103.5 113.03,109.22 C18.+ | v106.05,108.27 110.49,108.27 C18.+ | v106.05,97.79 R24.1 107.63,90.81 C12.1 IC1.12 | 119.7,107.63 R39.2 | IC3.7 187.64,92.71 186.69,91.76 186.69,90.49 185.1,88.9 180.98,88.9 C14.1 | 167.96,67.31 D28.A
  Bottom 1.422: v146.69,102.24 156.21,102.24 156.84,101.92 167.32,101.92 171.77,101.92 173.04,100.65 173.04,97.79 175.9,94.93 C14.1 R4.2
  Bottom 2.54: 99.06,115.25 96.84,117.44 TR1.PZ 96.73,116.84 99.06,115.25 | C18.+ 111.44,111.12 104.46,111.12 C28.1 99.06,110.17 | D7.C 99.06,110.17 | 99.06,110.17 99.06,115.25
GND  (via drill 0.6 pad 1.42, 0.6 pad 1.78)
  Top 0.305: v121.6,83.5 v121.6,90.49 | v141.92,68.58 v141.92,73.03
  Top 0.406: v69.21,130.49 v69.21,114.3 | 120.97,19.05 120.97,23.81 125.41,28.26 125.41,53.02 126.68,54.29 v126.68,66.04
  Top 1.676: PAD4.1 128.27,26.35 120.97,19.05
  Bottom 0.305: 121.6,91.12 121.6,92.08
  Bottom 0.813: 201.31,103.5 SV3.2 | IC1.1 124.14,79.69 121.6,82.23 v121.6,83.5 | 117.79,87.31 121.6,91.12
  Bottom 1.27: 124.42,79.65 IC1.1 | 183.5,109.24 183.83,108.9 | IC1.7 124.14,94.93 arc90 121.6,93.03 121.6,91.12 v121.6,90.49 | 117.79,87.31 IC1.13 | v69.21,130.49 59.69,140.02 57.79,140.02 53.92,143.88 TR3.1 | 201.3,108.9 SV3.2 201.28,98.44 R40.2 197.17,98.43 IC3.4 | D20.A 130.49,66.04 v126.68,66.04
  Bottom 1.422: 166.69,107.97 SV4.1 | SV1.3 110.21,70.13 R51.1
  Bottom 1.676: Q5.S 97.16,100.97
  Bottom 1.778: 76.83,80.96 R3.E 80.96,80.33 77.47,80.33
  Bottom 1.93: 133.67,109.85 132.08,111.44 132.08,116.91 TR2.P3
  Bottom 2.54: 168.59,108.9 R31.2 183.83,108.9 201.3,108.9 202.82,108.9 K1.1 | 167.32,107.63 165.74,107.63 | 97.16,100.97 101.28,105.09 C28.2 C18.-
  pour Bottom (isolate 1.27, no thermals): 118.74,41.27 118.74,34.92 131.13,34.92 131.13,41.27
  pour Bottom (isolate 1.27, no thermals): 118.11,118.11 132.72,118.11 132.72,113.66 132.72,113.03 119.38,113.03 117.47,114.94 117.47,118.11
  pour Bottom (isolate 1.016, no thermals): 176.85,87 176.85,114.94 176.21,115.25 121.92,115.57 108.27,102.55 102.55,102.55 98.11,98.11 87.95,98.11 87.95,115.25 67.94,115.25 67.94,83.82 72.39,79.38 94.93,79.38 100.33,73.98 100.33,62.23 169.55,62.23 169.55,79.38
N$1
  pour Bottom (no thermals): 154.94,124.46 173.36,124.46 173.36,146.05 157.48,146.05 157.48,130.18 154.94,127.63
N$2
  pour Bottom (no thermals): 178.44,146.05 178.44,124.46 186.69,124.46 186.69,132.72 191.14,137.16 191.14,146.05
N$3
  pour Bottom (isolate 1.016, no thermals): 183.52,175.26 179.71,175.26 179.71,168.91 175.9,165.1 166.37,165.1 166.37,163.2 177.17,163.2 179.07,165.1 190.5,165.1 194.31,161.29 194.31,160.02 191.14,156.84 178.44,156.84 178.44,149.86 195.58,149.86 195.58,113.03 198.12,113.03 198.12,161.29 189.23,170.18 arc-90
N$4
  Bottom 1.778: TR2.P1 142.74,125.41 C17.1 125.73,125.73 R29.2
  pour Bottom (no thermals): 146.69,155.57 146.69,146.05 141.61,146.05 141.61,139.06 144.78,139.06 144.78,128.27 149.86,128.27 153.35,131.44 153.35,149.54 153.99,150.18 153.99,152.4 150.5,155.57
N$5
  Bottom 1.422: 166.69,112.08 166.37,111.76 SV4.2 163.22,112.08 188.28,112.08 190.82,114.62 190.82,116.9 K1.2
  Bottom 2.54: D14.C C19.+ 163.22,112.08 166.69,112.08
N$6
  pour Bottom (isolate 1.016, no thermals): 164.47,177.17 164.47,170.18 173.36,170.18 173.36,179.71 193.68,179.71 193.68,173.99 203.84,163.83 203.84,127 201.3,127 201.3,161.93 191.14,172.09 187.33,175.26 187.33,177.17 175.9,177.17 175.9,168.91 174.62,167.64 161.93,167.64 161.93,177.17
N$7
  Bottom 0.813: R15.2 136.21,86.04 129.22,86.04 127.95,87.31 IC1.4
  Bottom 1.27: D3.C D2.C R15.2
N$8
  Bottom 2.54: TR2.P4 D14.A
N$9
  Bottom 1.778: L1.2 9.48,84.45 7.94,84.45 6.03,86.36 D27.A
N$10  (via drill 0.6 pad 1.93)
  Top 0.406: v108.9,94.93 v100.01,94.93
  Bottom 1.27: IC1.9 IC1.10 v108.9,94.93 | v100.01,94.93 R23.1 Q5.G
N$11
  Bottom 1.27: 151.55,43.18 D29.C 155.87,43.16 155.21,43.81 154.31,43.81 R49.2 | D26.C 150.69,41.91
  Bottom 2.54: Q11.G 150.69,41.91 150.69,42.32 151.55,43.18
N$13
  Bottom 1.27: R35.1 193.99,100.01 193.99,96.2 194.95,95.25 IC3.3 201.93,95.25 203.2,93.98 R40.1
N$14  (via drill 0.6 pad 2.18)
  Top 0.406: v93.66,80.96 86.36,73.66 86.36,28.89 106.05,9.21 136.21,9.21 141.92,14.92 141.92,18.73 141.61,19.05
  Top 1.676: PAD5.1 134.94,25.72 141.61,19.05
  Bottom 1.27: R2.A v93.66,80.96 | D26.A 140.02,38.04 Q11.S
  Bottom 1.676: PAD5.1 139.51,37.47 Q11.S
N$15
  Bottom 2.54: D8.C D9.C
N$16
  Bottom 1.27: R52.1 93.98,85.09 93.03,86.04 C30.1
  Bottom 1.422: R2.S R2.E 93.03,86.04
N$17  (1 unrouted)
  Bottom 1.27: 104.14,85.18 R52.2 | IC1.16 R51.2 105.5,79.69 104.25,80.94 R52.2 | C30.2 100.65,87.63 103.21,85.07 R52.2
N$18
  Bottom 0.813: IC1.5 D5.C
  Bottom 1.27: D5.C C9.2
N$19
  Bottom 0.813: R19.2 IC1.6
N$20
  Bottom 1.93: R21.2 D6.C R17.2 75.88,98.11 R14.1
N$21  (via drill 0.6 pad 2.18)
  Top 0.406: v73.34,130.81 v73.34,116.52
  Bottom 0.305: R21.1 73.34,114.62
  Bottom 1.27: v73.34,116.52 73.34,114.62 | v73.34,130.81 58.9,145.26 TR3.2
  Bottom 1.93: R21.1 D6.A
N$22
  Bottom 0.813: IC1.8 119.06,97.47 119.06,92.39 IC1.11
  Bottom 1.27: R24.2 IC1.11
N$23
  Bottom 1.27: Q5.D 93.98,102.87
  Bottom 2.54: 86.38,117.49 TR1.PK 83.82,114.88 D7.A 85.72,107.95 90.49,107.95 93.98,104.46 93.98,102.87
N$24
  Bottom 1.422: R28.2 Q7.B
N$25
  Bottom 1.27: D23.C D24.A
N$26
  Bottom 1.778: TR1.S1Z 85.88,144 83.82,146.05 74.93,146.05 69.21,151.77 R28.1
  Bottom 1.93: R28.1 D11.A
N$27
  pour Bottom (isolate 1.016, no thermals): 47.62,161.29 47.62,165.74 52.07,165.74 54.61,163.2 57.15,163.2 57.15,161.29
N$28
  Bottom 1.27: R27.2 Q6.B
N$29
  Bottom 1.27: TR1.S2Z 106.05,135.78 106.05,132.72 103.5,130.18 79.69,130.18 75.56,126.05 10.79,126.05 5.71,130.81 D10.A R27.1
N$30
  Bottom 1.27: 67.56,175.51 D21.C
  pour Bottom (isolate 1.016, no thermals): 37.47,143.51 37.47,148.91 45.09,157.48 54.61,157.48 55.25,156.84 58.42,156.84 59.69,158.12 59.69,177.17 69.21,177.17 69.21,173.99 65.41,173.99 65.41,151.13 73.66,142.88 82.55,142.88 82.55,137.79 75.56,137.79 61.59,151.77 51.44,151.77 49.21,149.54 49.21,143.51
N$31
  pour Bottom (isolate 1.016, no thermals): 6.35,149.86 3.81,149.86 3.81,165.1 6.35,165.1
N$32
  pour Bottom (isolate 1.016, no thermals): 156.84,177.17 156.84,170.81 154.31,168.91 151.13,168.91 141.61,159.39 152.4,159.39 157.48,154.31 157.48,149.86 173.36,149.86 173.36,156.84 175.9,159.39 175.9,161.29 164.47,161.29 159.39,166.37 159.39,177.17
N$33
  Bottom 1.93: D8.A IC2.5
  Bottom 2.184: TR2.P2 128.59,132.9 D8.A
N$34
  Bottom 1.27: IC2.1 C15.1
N$35
  Bottom 1.27: IC2.4 R29.1 OK1.4
N$36
  Bottom 1.27: D22.C 1.91,61.59 0.64,62.87 0.64,76.2 3.81,79.38 | 9.48,79.38 L1.1
  Bottom 1.778: 3.81,79.38 3.85,79.41 L1.1
  pour Bottom (isolate 1.27, no thermals): 3.17,63.5 3.17,59.69 9.21,59.69 11.11,57.78 22.54,57.78 22.54,66.04 11.43,66.04 9.21,63.5
N$37
  Bottom 2.54: D15.A 142.88,114.62 145.34,117.08 TR2.P5
N$38
  Bottom 1.27: 14.29,166.05 15.88,167.64 15.88,172.4 16.83,173.36
  Bottom 2.184: 16.83,173.36 18.22,174.75 Q8.G
  Bottom 2.54: R36.2 14.29,166.05
N$39
  pour Bottom (isolate 1.016, no thermals): 19.68,143.51 19.68,153.35 21.91,155.57 21.91,177.8 25.08,177.8 25.08,162.24 30.48,156.84 36.83,156.84 41.59,161.61 41.59,177.17 43.82,177.17 43.82,159.7 34.29,150.18 34.29,143.51
N$40
  Bottom 1.27: OK1.1 115.57,114.94 116.84,113.66 R38.2 118.74,112.71 D16.A
N$41
  Bottom 1.27: R39.1 128.59,108.27 D16.C
N$42
  Bottom 2.54: R37.2 50.16,173.36 50.16,175.9 50.29,175.13 Q9.G
N$43
  Bottom 1.27: R1.2 140.65,99.83 D2.A 146.05,94.93 146.37,95.25 R26.S R26.E C1.-
N$44
  Bottom 1.27: R41.1 19.37,163.11 C20.1 D18.A
N$45
  pour Bottom (isolate 1.016, no thermals): 67.94,164.47 67.94,171.77 70.48,171.77 70.48,164.47
N$46
  Bottom 1.27: R30.2 R35.2 184.15,101.28 185.1,100.33 190.18,100.33 191.45,99.06 191.45,95.88 190.82,95.25 IC3.6
N$47
  pour Bottom (isolate 1.27, no thermals): 3.49,66.04 3.49,74.93 12.38,74.93 18.73,81.28 18.73,102.55 39.05,102.55 39.05,68.58 11.11,68.58 8.57,66.04
N$48
  Bottom 1.27: D24.C 163.51,35.56
  Bottom 1.778: 163.51,35.56 165.42,37.47 R62.1
  Bottom 2.54: C26.+ 95.88,48.89 | R25.1 R13.1 R61.1 169.07,48.1 | 169.07,48.1 168.91,47.94 145.1,47.94 | 169.07,48.1 169.07,42.7 R62.1
  pour Bottom (no thermals): 57.15,64.45 97.16,64.45 97.16,55.88 103.82,49.21 147,49.21 147,35.56 143.19,35.56 143.19,43.81 141.92,45.09 132.08,45.09 130.81,43.81 101.28,43.81 98.11,46.99 57.15,46.99
N$49
  Bottom 0.813: IC1.2 125.41,82.23 130.81,76.84 D20.C | IC3.2 200.03,92.71 200.98,91.76 200.98,87.63 196.85,83.5 177.48,83.5 175.9,81.91 172.72,81.91 169.86,79.06 169.86,63.82 167.96,61.91 160.66,61.91 154.31,68.26
  Bottom 1.27: 147.64,68.26 146.82,68.26 R8.2 144.28,70.8 C7.2 134.94,70.8 130.81,74.93 D20.C | 147.64,68.26 154.31,68.26 | R43.1 147.64,68.26
N$50
  Bottom 1.27: D3.A 151.45,84.45 R12.2 D1.C | D1.C 153.99,84.77 D3.A | D3.A 151.77,87 Q2.C 155.89,86.04 D1.C
N$51  (via drill 0.6 pad 1.78)
  Top 0.406: v105.73,55.88 v105.73,41.27
  Bottom 0.813: 147.77,55.88 R43.2 147.64,55.88 147.77,55.88
  Bottom 1.27: v105.73,55.88 R47.1 112.71,55.88 115.25,58.42 Q10.E 131.45,58.42 133.99,55.88 147.51,55.88 R43.2
  Bottom 1.778: v105.73,41.27 110.81,41.27 R44.1
  Bottom 2.54: R44.1 112.39,34.92 116.2,31.12 185.74,31.12 189.87,35.24 189.87,41.08
  pour Bottom (isolate 1.27, no thermals): 59.69,102.55 59.69,81.91 68.9,72.71 94.93,72.71 97.16,70.48 97.16,67.63 53.34,67.63 53.34,43.81 96.52,43.81 99.69,40.96 102.87,40.96 104.77,39.05 110.81,39.05 110.81,41.27 115.25,41.27 115.25,29.21 15.56,29.21 15.56,40.96 11.43,45.09 3.49,45.09 3.49,57.15 8.57,57.15 10.16,55.56 40.01,55.56 41.91,57.47 41.91,102.55
  pour Bottom (isolate 1.27, no thermals): 172.72,58.1 172.72,78.11 173.67,79.06 176.85,79.06 179.07,81.28 209.55,81.28 209.55,48.58 189.87,29.21 111.12,29.21 111.12,36.2 115.25,36.2 115.25,32.38 170.18,32.38 188.28,50.48 202.25,50.48 202.25,58.1
N$52
  Bottom 1.27: SV2.1 142.6,60.05 141.61,60.09 138.43,63.18 R53.S R53.A
  Bottom 1.676: 136.53,65.72 R53.A
N$53
  Bottom 1.27: SV2.2 144.28,62.55 R8.1 144.09,62.55 C36.1
N$54
  Bottom 0.813: IC1.15 117.16,82.23 119.38,80.01 119.38,74.93 C6.2
  Bottom 1.27: R5.1 IC1.15
N$55
  Bottom 1.27: R5.2 SV1.2
N$56
  Bottom 1.27: R47.2 R46.1 Q10.B
N$57
  Bottom 1.676: R59.2 15.24,4.45 16.83,2.86 26.99,2.86 29.84,5.71 PAD7.1 PAD12.1
  pour Bottom (isolate 1.016, no thermals): 15.88,5.4 0.95,5.4 0.95,11.43 15.88,11.43
N$58
  Bottom 1.27: C6.1 R10.2
N$59
  Bottom 1.27: Q2.B 160.02,89.53 R6.1
N$60
  Bottom 1.27: Q13.1 17.89,15.35 18.1,15.56
  Bottom 2.54: 18.1,15.56 22.22,19.69 R58.1 R57.2 PAD6.1 PAD13.1
N$61
  Bottom 1.27: R6.2 Q3.C | R6.2 Q1.C | R4.1 R6.2
N$62
  Bottom 1.27: SV5.1 4.74,12.7 19.68,12.7 Q13.3 23.28,12.7 31.11,12.7 33.02,10.8 R57.1
N$63
  Bottom 1.27: Q4.E 145.42,82.23 146.69,80.96 R9.2 R7.1 159.07,79.69 Q3.B
N$64
  Bottom 1.27: R34.E 184.15,96.84 185.1,97.79 IC3.5
N$65
  Bottom 0.61: IC3.1 195.26,90.17 191.45,93.98 186.37,93.98 184.15,91.76
  Bottom 1.27: 184.15,91.76 R34.A
N$66
  Bottom 1.27: IC1.3 127.64,84.77 R10.1 138.43,84.14 R11.1
N$67
  Bottom 1.27: Q10.C 149.64,53.34 R49.1 150.87,53.34 R48.2
N$68
  Bottom 0.813: 181.61,94.3 179.39,96.52 R31.1
  Bottom 1.27: 181.61,94.3 R34.S
N$69
  Bottom 1.27: C7.1 R11.2
N$70
  Bottom 0.813: C37.+ 71.09,75.56 95.25,75.56 99.69,71.12 99.69,57.15 105.73,51.12 160.34,51.12 R48.1
  Bottom 1.27: D27.C 6.03,103.19 12.06,109.22 60.64,109.22 64.77,105.09 64.77,81.91 C37.+ | R48.1 D28.C
N$71
  Bottom 1.27: C3.1 R14.2 R3.A
N$72
  pour Bottom (isolate 1.016, no thermals): 189.87,161.93 189.87,159.39 180.98,159.39 180.98,161.93
N$73  (via drill 0.6 pad 1.78)
  Top 0.406: v159.07,70.48 v159.07,58.1
  Bottom 0.813: v159.07,58.1 134.62,58.1 132.4,60.33 103.5,60.33 102.23,61.59 102.23,72.39 96.52,78.11 86.04,78.11 84.45,79.69 84.45,81.91 82.87,83.5 R3.S
  Bottom 1.27: Q1.B v159.07,70.48
N$74
  Bottom 1.27: R30.1 197.19,105.73 SV3.1
N$75
  Bottom 1.422: Q13.2 17.99,10.9 17.78,10.8 R59.1
  pour Bottom (isolate 1.016, no thermals): 17.14,7.62 17.14,11.11 28.57,10.8 30.16,9.21 30.16,7.62
N$76
  Bottom 1.27: C32.2 R60.1 56.52,8.89 58.1,10.48 66.04,10.48 67.31,9.21 67.31,7.62 Q12.2
N$77
  Bottom 1.27: TR4.P R60.2 71.12,3.18 Q12.3
N$78
  Bottom 1.27: D25.C 71.12,20 C33.+ 73.34,19.05 PAD9.1
N$79
  Bottom 1.27: R9.1 D1.A
N$80
  Bottom 1.27: R18.2 131.45,79.69 D5.A | D5.A D4.A | D5.A Q4.B
N$81
  Bottom 0.406: R45.1 C23.1
N$82
  Bottom 1.27: TR4.S2 68.26,17.46 69.21,16.51 C33.- 72.07,15.24 78.1,9.21 PAD8.1
N$83
  Bottom 1.27: TR4.I C32.1
N$84
  Bottom 1.27: PAD11.1 45.72,10.16 50.8,10.16 52.07,8.89 TR4.SP
N$85
  Bottom 1.27: Q12.1 66.04,13.97 44.13,13.97 PAD10.1
N$86
  Bottom 1.27: TR4.S1 51.44,20 D25.A
N$87
  Bottom 0.305: 26.04,183.83 -0.32,183.83 -0.32,120.97
N$88
  Bottom 0.305: 193.68,29.21 209.55,29.21 209.55,44.77
N$89
  Bottom 0.305: 209.55,183.83 209.55,130.18
N$90
  Bottom 0.305: 209.55,183.83 177.8,183.83
N$91
  Bottom 0.305: 0,39.05 0,29.21 13.34,29.21
N$92
  Bottom 0.305: 209.55,107.63 209.55,86.04
N$93
  Bottom 1.27: D29.A D23.A
V+  (via drill 0.8 pad 1.93)
  Top 0.305: v138.43,153.67 v138.43,172.72
  Bottom 1.27: v138.43,172.72 138.43,172.28
  Bottom 2.54: D17.C 37.47,180.66 | 55.88,178.44 Q9.D R42.2 D19.A | R22.1 137.48,152.72 v138.43,153.67
  Bottom 3.81: 55.88,181.61 55.88,178.44
  Bottom 5: 81.91,176.53 81.91,181.61 55.88,181.61 36.2,181.61
  pour Bottom (isolate 0.61, no thermals): 146.69,179.71 167,179.71 167,172.72 170.18,172.72 170.18,183.83 79.38,183.83 79.38,173.36 88.9,163.83 130.81,163.83
  pour Bottom (isolate 1.016, no thermals): 33.66,183.83 33.66,170.18 34.93,168.91 38.73,168.91 39.05,183.83
  pour Bottom (no thermals): 136.53,149.22 136.53,153.03 139.06,155.57 143.51,155.57 143.51,149.22
V-  (via drill 0.6 pad 1.93, 0.6 pad 2.18, 0.9 pad 2.18)
  Top 0.406: v32.7,160.02 v15.24,160.02
  Top 1.27: v76.2,151.77 43.18,151.77 v36.2,160.66
  pour Bottom (isolate 1.27, no thermals): 132.72,159.39 88.9,159.39 76.2,172.09 76.2,177.17 73.02,177.17 73.02,173.36 74.3,170.18 74.3,153.03 76.2,150.5 86.36,150.5 90.17,146.69 97.79,146.69 99.69,144.78 99.69,137.79 102.87,137.79 102.87,144.78 104.77,146.69 117.47,146.69 117.47,140.34 111.12,140.34 111.12,136.53 117.47,136.53 117.47,124.46 120.02,124.46 120.02,136.53 123.19,139.06 137.8,139.06 137.8,146.05 132.72,146.05 132.72,154.31 151.13,172.72 154.31,172.72 154.31,177.17 150.5,177.17
  pour Bottom (no thermals): 38.73,161.93 38.73,166.37 33.34,166.37 31.43,168.28 31.43,177.8 27.62,177.8 27.62,163.83 32.07,159.39 36.2,159.39
  pour Bottom (isolate 1.27, no thermals): 10.79,161.93 10.79,154.31 16.51,154.31 16.51,160.97 15.56,161.93
(copper drawn outside any net)
  shapes: Bottom area x5, Bottom circle x8, Top circle x2

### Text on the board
Top: +17V
Bottom: LED | FAN | +
tPlace: 140z | 16z | 7z | 17v | ukostrenie folie | 12v | ventilator | LED obm. prudu | duty cycle 0,45 | nast. indikacie obm.prudu | nast.napetia | šp.prud | pot. napetie | E | Max. prud | B | pot. prud | C | (2SC2610 osadit opacne) | 1u/100 | P6.. | gnd | DC to DC | cerveny | cerveny | 12V | Hfe=160 | +12v | +12v | 4.5-30V | modul TK1382 | modry | Converter | V+ | stred | ak je pouzity bocnik | Rb | A | V | meriame az zanim | cierny | 4.5-30V | cierny | kraj
Document: ~230V | -80v | +80V
hacesoft: oblasti ktore treba hrubo pocinovat
separator: Chladic a bezpecnostna medzera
